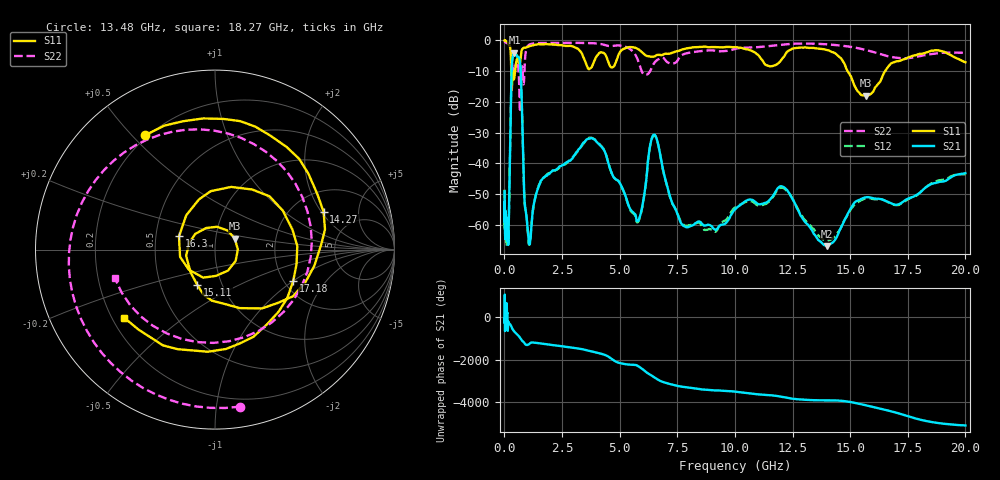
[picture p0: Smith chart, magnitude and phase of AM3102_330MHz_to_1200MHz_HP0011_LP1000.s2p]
! Date/Time: Tue, Sep 11, 2018 5:12 PM
! Network Analyzer: Agilent Technologies E8362B Rev: A.07.50.63
! Sweep from 0.010 to 20.000 GHz, 1601 Points, Sweep Type: LOG
! Power Supply: 4.950 V, 0.001 A
# Hz S DB R 50
!freq MagS11 AngS11 MagS21 AngS21 MagS12 AngS12 MagS22 AngS22
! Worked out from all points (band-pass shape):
!   1601 points, 10 MHz to 20 GHz, reference 50 ohm
!   highest |S21| = -3.96 dB at 434.6 MHz (marker M1); lowest = -66.9 dB at 14.01 GHz (marker M2)
!   |S21| within 3 dB of the highest: 333.4 MHz to 675.6 MHz (342.2 MHz wide, 67.8 % of centre)
!   lowest |S11| = -18.0 dB at 15.7 GHz (marker M3), VSWR 1.29, Z = 61.9 + j7.63 ohm
!   |S11| at or under -10 dB: 299 MHz to 359.5 MHz (60.44 MHz wide, 18.4 % of centre); 366.7 MHz to 469.2 MHz (102.6 MHz wide, 24.5 % of centre); 14.89 GHz to 16.52 GHz (1.622 GHz wide, 10.3 % of centre)
!   |S22| runs from -23.4 to -0.3 dB; largest |S21 - S12| = 0.012
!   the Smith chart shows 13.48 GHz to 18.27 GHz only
!   S11 on the Smith chart (normalised r, x): 13.48 GHz: 0.19, +0.55; 14.27 GHz: 2.95, +2.10; 15.11 GHz: 0.76, -0.31; 16.3 GHz: 0.66, +0.10; 17.18 GHz: 2.24, -1.00; 18.27 GHz: 0.25, -0.32
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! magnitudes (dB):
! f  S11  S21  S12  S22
! 10 MHz  0.0  -49.1  -48.5  -0.3
! 35.55 MHz  0.0  -63.8  -63.4  -0.5
! 126.4 MHz  -0.4  -64.4  -63.0  -0.9
! 182.2 MHz  -1.0  -61.5  -62.7  -1.2
! 434.6 MHz  -11.9  -4.0  -4.0  -9.9
! 447.2 MHz  -11.1  -4.0  -4.0  -9.3
! 689.1 MHz  -6.8  -8.0  -8.1  -22.8
! 1.072 GHz  -1.9  -66.3  -66.2  -1.4
! 1.59 GHz  -1.3  -45.6  -45.8  -0.8
! 3.793 GHz  -8.6  -31.8  -31.7  -0.9
! 5.652 GHz  -2.3  -56.4  -56.7  -4.3
! 6.518 GHz  -5.2  -30.6  -30.8  -7.1
! 7.845 GHz  -2.7  -60.6  -60.3  -4.3
! 13.48 GHz  -2.5  -63.4  -62.1  -1.0
! 14.01 GHz  -3.1  -66.9  -65.2  -1.3
! 14.27 GHz  -3.9  -65.6  -64.2  -1.4
! 15.11 GHz  -13.2  -53.6  -54.1  -2.2
! 15.7 GHz  -18.0  -51.0  -51.4  -3.1
! 16.3 GHz  -13.4  -51.6  -51.7  -4.4
! 17.18 GHz  -6.6  -53.1  -53.3  -5.7
! 18.27 GHz  -4.0  -47.8  -47.8  -4.7
! 20 GHz  -7.1  -43.2  -43.6  -4.0
